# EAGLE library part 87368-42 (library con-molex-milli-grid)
RECEPTACAL
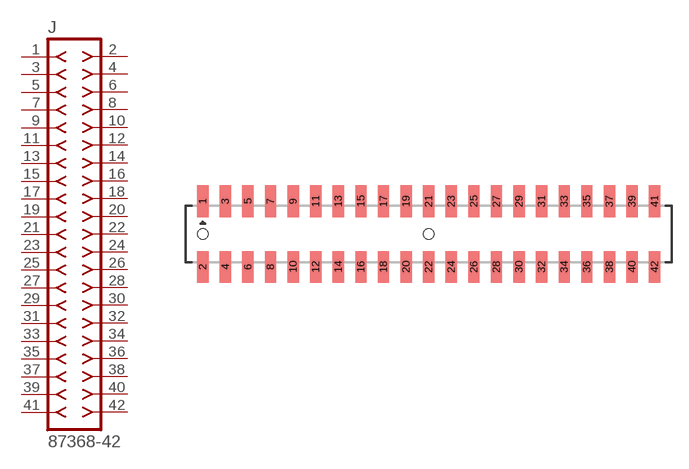
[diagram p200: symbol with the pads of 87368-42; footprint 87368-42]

Designator prefix J

## 87368-42  [87368-42]
1  1  pas
2  2  pas
3  3  pas
4  4  pas
5  5  pas
6  6  pas
7  7  pas
8  8  pas
9  9  pas
10  10  pas
11  11  pas
12  12  pas
13  13  pas
14  14  pas
15  15  pas
16  16  pas
17  17  pas
18  18  pas
19  19  pas
20  20  pas
21  21  pas
22  22  pas
23  23  pas
24  24  pas
25  25  pas
26  26  pas
27  27  pas
28  28  pas
29  29  pas
30  30  pas
31  31  pas
32  32  pas
33  33  pas
34  34  pas
35  35  pas
36  36  pas
37  37  pas
38  38  pas
39  39  pas
40  40  pas
41  41  pas
42  42  pas

## Footprint 87368-42 (pad centres in mm)
RECEPTACAL SMD Dual Row, Side Entry
smd 1 x 2.8: 1 -20,2.9; 2 -20,-2.9; 3 -18,2.9; 4 -18,-2.9; 5 -16,2.9; 6 -16,-2.9; 7 -14,2.9; 8 -14,-2.9; 9 -12,2.9; 10 -12,-2.9; 11 -10,2.9; 12 -10,-2.9; 13 -8,2.9; 14 -8,-2.9; 15 -6,2.9; 16 -6,-2.9; 17 -4,2.9; 18 -4,-2.9; 19 -2,2.9; 20 -2,-2.9; 21 0,2.9; 22 0,-2.9; 23 2,2.9; 24 2,-2.9; 25 4,2.9; 26 4,-2.9; 27 6,2.9; 28 6,-2.9; 29 8,2.9; 30 8,-2.9; 31 10,2.9; 32 10,-2.9; 33 12,2.9; 34 12,-2.9; 35 14,2.9; 36 14,-2.9; 37 16,2.9; 38 16,-2.9; 39 18,2.9; 40 18,-2.9; 41 20,2.9; 42 20,-2.9
hole 0.914 at -20,0
hole 0.914 at 0,0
